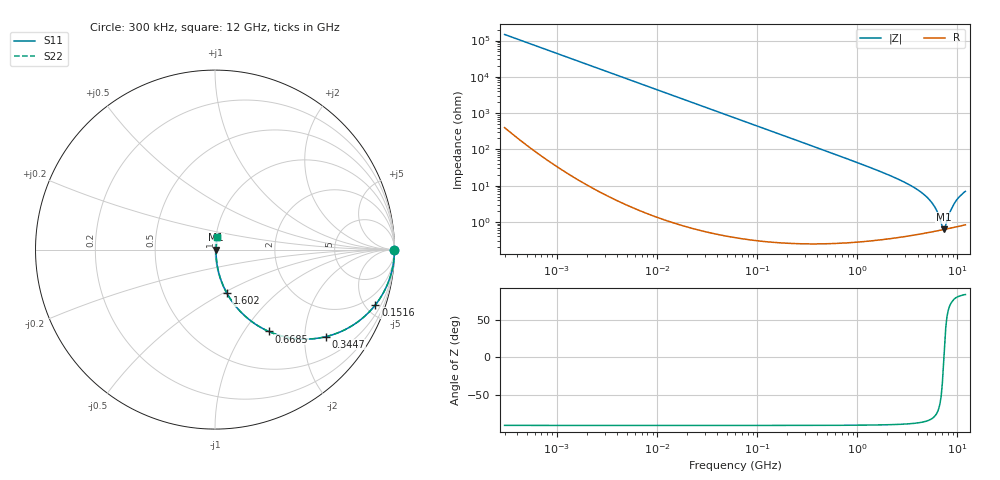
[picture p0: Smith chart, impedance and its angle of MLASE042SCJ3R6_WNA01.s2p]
! MLASE042SCJ3R6_WNA01  S-PARAMETER MODEL  ( General Type )
! Model Generated by TAIYO YUDEN Corporation (http://www.ty-top.com)
! Version 1.0
! TAIYO YUDEN Control No. 120810
! Copyright(c) 2012 TAIYO YUDEN CO.,LTD. All Rights Reserved.
! Product Description (link to TY-COMPAS)
! https://ds.yuden.co.jp/TYCOMPAS/or/detail?pn=MLASE042SCJ3R6BWNA01&u=M
! Products Name : Multilayer Ceramic Capacitors
! Characteristics :
!  Capacitance : 3.6 pF , Rated Voltage : 16V , TCC : CJ / C0J
!  Case Size : 0.4 x 0.2 / 0.016 x 0.008 [mm/inch] , Thickness : 0.2 / 0.008 [mm/inch]
!  (Conditions: Temperature = 25 degC , DC Bias Current/Voltage = 0A / 0V)
! External Node Assignments :
!  1  o---| |---o  2
! GND o---------o GND
! Frequency Range : 0.3MHz  -  12000MHz  [ 401 STEP ]
# MHz S RI R 50
! Freq[MHz].  S11 Real  S11 Imag  S21 Real  S21 Imag  S12 Real  S12 Imag  S22 Real  S22 Imag
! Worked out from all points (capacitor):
!   401 points, 300 kHz to 12 GHz, reference 50 ohm
!   read as one part in series: C = 3.62 pF near 316.3 kHz
!   lowest |Z| = 622 mohm at 7.254 GHz (marker M1)
!   series resonance near 7.313 GHz, so ESL is about 130 pH
!   S11 on the Smith chart (normalised r, x): 300 kHz: open; 151.6 MHz: 1.01, -5.80; 344.7 MHz: 1.00, -2.55; 668.5 MHz: 1.01, -1.31; 1.602 GHz: 1.01, -0.52; 12 GHz: 1.02, +0.14
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0.3  1 -0.000682  2.31e-06 0.000682  2.31e-06 0.000682  1 -0.000682
1.769972  1 -0.00402  1.82e-05 0.00402  1.82e-05 0.00402  1 -0.00402
10.44266  0.9994 -0.0237  0.00057 0.0237  0.00057 0.0237  0.9994 -0.0237
60  0.9817 -0.1339  0.0183 0.1339  0.0183 0.1339  0.9817 -0.1339
151.6462  0.8935 -0.308  0.1065 0.308  0.1065 0.308  0.8935 -0.308
225.6362  0.7911 -0.4059  0.2089 0.4059  0.2089 0.4059  0.7911 -0.4059
344.7396  0.6182 -0.4848  0.3818 0.4848  0.3818 0.4848  0.6182 -0.4848
353.9943  0.6056 -0.4877  0.3944 0.4877  0.3944 0.4877  0.6056 -0.4877
668.5285  0.2994 -0.456  0.7006 0.456  0.7006 0.456  0.2994 -0.456
1021.415  0.153 -0.3567  0.847 0.3567  0.847 0.3567  0.153 -0.3567
1602.47  0.0665 -0.2432  0.9335 0.2432  0.9335 0.2432  0.0665 -0.2432
2088.533  0.0391 -0.1852  0.9609 0.1852  0.9609 0.1852  0.0391 -0.1852
3454.93  0.0138 -0.0971  0.9862 0.0971  0.9862 0.0971  0.0138 -0.0971
4875.354  0.00741 -0.0495  0.9926 0.0495  0.9926 0.0495  0.00741 -0.0495
6026.253  0.00605 -0.0231  0.9939 0.0231  0.9939 0.0231  0.00605 -0.0231
6879.757  0.00598 -0.00721  0.994 0.00721  0.994 0.00721  0.00598 -0.00721
7254.098  0.00611 -0.000928  0.9939 0.000928  0.9939 0.000928  0.00611 -0.000928
7648.807  0.00632 0.00532  0.9937 -0.00532  0.9937 -0.00532  0.00632 0.00532
8503.825  0.00704 0.0185  0.993 -0.0185  0.993 -0.0185  0.00704 0.0185
9454.42  0.00826 0.0335  0.9917 -0.0335  0.9917 -0.0335  0.00826 0.0335
10511.28  0.01 0.0487  0.99 -0.0487  0.99 -0.0487  0.01 0.0487
12000  0.0129 0.0677  0.9871 -0.0677  0.9871 -0.0677  0.0129 0.0677
